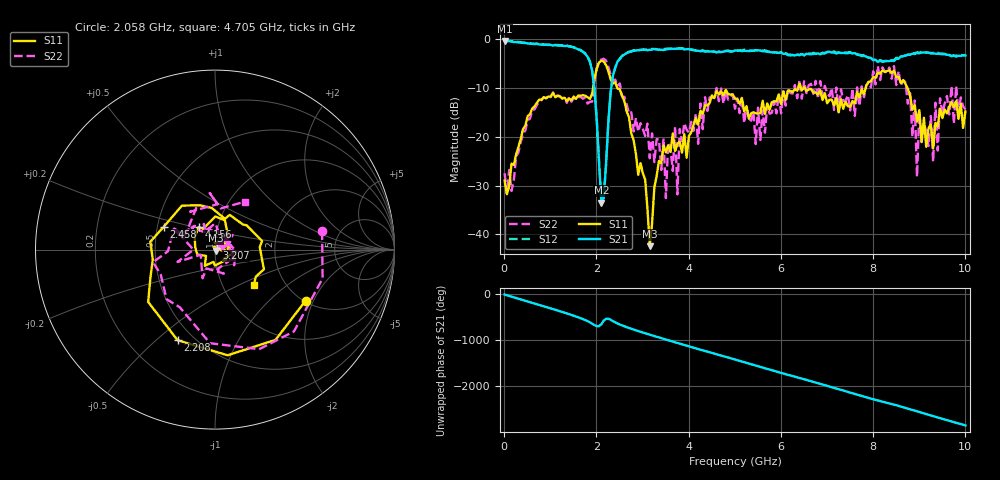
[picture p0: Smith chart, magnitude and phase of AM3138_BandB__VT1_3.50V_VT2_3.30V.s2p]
! Date/Time: Tue, Nov 13, 2018 4:39 PM
! Network Analyzer: Agilent Technologies E8364B Rev: A.07.50.67
! Sweep from 0.010 to 10.000 GHz, 201 Points, Sweep Type: LIN
! Power Supply: 3.501 V, 0.000 A
# Hz S DB R 50
!freq MagS11 AngS11 MagS21 AngS21 MagS12 AngS12 MagS22 AngS22
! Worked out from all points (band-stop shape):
!   201 points, 10 MHz to 10 GHz, reference 50 ohm
!   highest |S21| = -0.31 dB at 10 MHz (marker M1); lowest = -33.5 dB at 2.108 GHz (marker M2)
!   |S21| within 3 dB of the highest: start of sweep to 1.786 GHz; 2.574 GHz to 6.302 GHz (3.728 GHz wide, 84 % of centre)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
!   lowest |S11| = -42.4 dB at 3.157 GHz (marker M3), VSWR 1.02, Z = 50.3 - j0.688 ohm
!   |S11| at or under -10 dB: start of sweep to 1.926 GHz; 2.454 GHz to 6.372 GHz (3.918 GHz wide, 88.8 % of centre); 6.519 GHz to 7.837 GHz (1.319 GHz wide, 18.4 % of centre)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
!   |S22| runs from -32.6 to -4.0 dB; largest |S21 - S12| = 0.028
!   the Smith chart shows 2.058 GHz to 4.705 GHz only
!   S11 on the Smith chart (normalised r, x): 2.058 GHz: 2.03, -1.74; 2.208 GHz: 0.41, -0.59; 2.458 GHz: 0.54, +0.15; 3.207 GHz: 1.02, +0.02; 4.156 GHz: 0.81, +0.21; 4.705 GHz: 1.40, -0.61
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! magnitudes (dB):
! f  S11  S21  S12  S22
! 10 MHz  -29.0  -0.3  -0.2  -27.5
! 1.708 GHz  -11.4  -2.6  -2.5  -12.2
! 2.058 GHz  -4.7  -25.3  -25.1  -4.4
! 2.108 GHz  -4.4  -33.5  -33.2  -4.1
! 2.208 GHz  -5.2  -25.9  -25.9  -4.3
! 2.458 GHz  -10.1  -4.6  -4.6  -9.6
! 3.157 GHz  -42.4  -2.2  -2.0  -24.4
! 3.207 GHz  -37.8  -2.1  -2.0  -19.3
! 3.357 GHz  -24.9  -2.1  -2.1  -20.6
! 3.507 GHz  -23.2  -2.1  -1.9  -32.6
! 3.706 GHz  -22.9  -1.9  -1.9  -17.9
! 3.756 GHz  -21.4  -1.9  -1.9  -31.8
! 3.806 GHz  -21.0  -1.9  -1.8  -18.4
! 4.156 GHz  -16.2  -2.3  -2.3  -15.2
! 4.705 GHz  -10.7  -2.6  -2.6  -10.1
! 5.005 GHz  -12.1  -2.3  -2.4  -14.2
! 6.703 GHz  -10.9  -3.0  -2.7  -11.2
! 8.352 GHz  -6.3  -4.5  -4.5  -5.8
! 8.901 GHz  -13.5  -3.0  -2.9  -12.5
! 8.951 GHz  -16.9  -2.8  -2.6  -28.2
! 9.001 GHz  -14.5  -2.9  -2.7  -14.9
! 10 GHz  -14.8  -3.3  -3.2  -14.4
